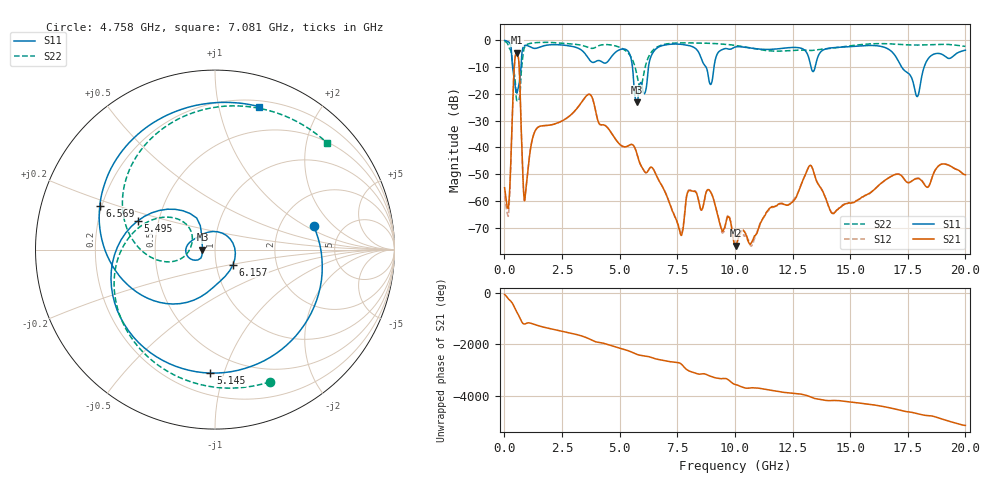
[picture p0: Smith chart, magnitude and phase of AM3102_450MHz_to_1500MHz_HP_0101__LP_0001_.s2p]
!Agilent Technologies,E8364B,MY43040894,A.07.50.67
!Agilent E8364B: A.07.50.67
!Date: Thursday, January 11, 2018 05:39:38
!Correction: S11(Full 2 Port(1,2))
!S21(Full 2 Port(1,2))
!S12(Full 2 Port(1,2))
!S22(Full 2 Port(1,2))
!S2P File: Measurements: S11, S21, S12, S22:
# Hz S  dB  R 50
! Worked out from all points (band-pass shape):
!   1601 points, 10 MHz to 20 GHz, reference 50 ohm
!   highest |S21| = -4.63 dB at 534.7 MHz (marker M1); lowest = -76.6 dB at 10.04 GHz (marker M2)
!   |S21| within 3 dB of the highest: 450.6 MHz to 622.9 MHz (172.3 MHz wide, 32.1 % of centre)
!   lowest |S11| = -23.1 dB at 5.745 GHz (marker M3), VSWR 1.15, Z = 43.5 + j0.00252 ohm
!   |S11| at or under -10 dB: 356.6 MHz to 722.1 MHz (365.5 MHz wide, 67.8 % of centre); 5.557 GHz to 6.249 GHz (692.5 MHz wide, 11.7 % of centre); 17.24 GHz to 18.21 GHz (973.1 MHz wide, 5.49 % of centre)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
!   |S22| runs from -22.6 to -0.4 dB; largest |S21 - S12| = 0.0032
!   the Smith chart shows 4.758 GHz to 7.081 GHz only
!   S11 on the Smith chart (normalised r, x): 4.758 GHz: 3.09, +1.20; 5.145 GHz: 0.34, -0.90; 5.495 GHz: 0.38, +0.15; 6.157 GHz: 1.20, -0.21; 6.569 GHz: 0.19, +0.18; 7.081 GHz: 0.25, +1.32
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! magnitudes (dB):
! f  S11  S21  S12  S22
! 10 MHz  -0.1  -55.0  -58.0  -0.4
! 197.4 MHz  -0.7  -60.5  -63.2  -2.6
! 534.7 MHz  -19.7  -4.6  -4.6  -22.4
! 897.1 MHz  -1.9  -58.6  -58.4  -2.2
! 1.384 GHz  -3.0  -33.1  -33.1  -0.9
! 3.346 GHz  -3.7  -23.1  -23.1  -1.8
! 4.758 GHz  -5.0  -36.1  -36.1  -2.0
! 5.145 GHz  -3.2  -39.6  -39.6  -3.2
! 5.495 GHz  -6.7  -38.9  -38.9  -6.2
! 5.745 GHz  -23.1  -42.2  -42.2  -12.8
! 6.157 GHz  -17.7  -49.4  -49.4  -8.4
! 6.569 GHz  -3.3  -50.0  -50.0  -2.8
! 6.682 GHz  -2.5  -52.0  -52.0  -2.3
! 7.081 GHz  -1.6  -58.9  -58.8  -1.3
! 8.943 GHz  -16.5  -56.6  -56.4  -1.1
! 10.01 GHz  -2.5  -76.2  -76.7  -1.9
! 10.04 GHz  -2.4  -76.6  -76.6  -1.9
! 13.34 GHz  -11.1  -47.3  -47.3  -3.8
! 14.25 GHz  -2.8  -64.6  -64.3  -2.9
! 16.68 GHz  -3.4  -51.3  -51.3  -1.3
! 17.9 GHz  -21.0  -51.6  -51.4  -1.8
! 20 GHz  -3.7  -50.2  -50.2  -2.3
